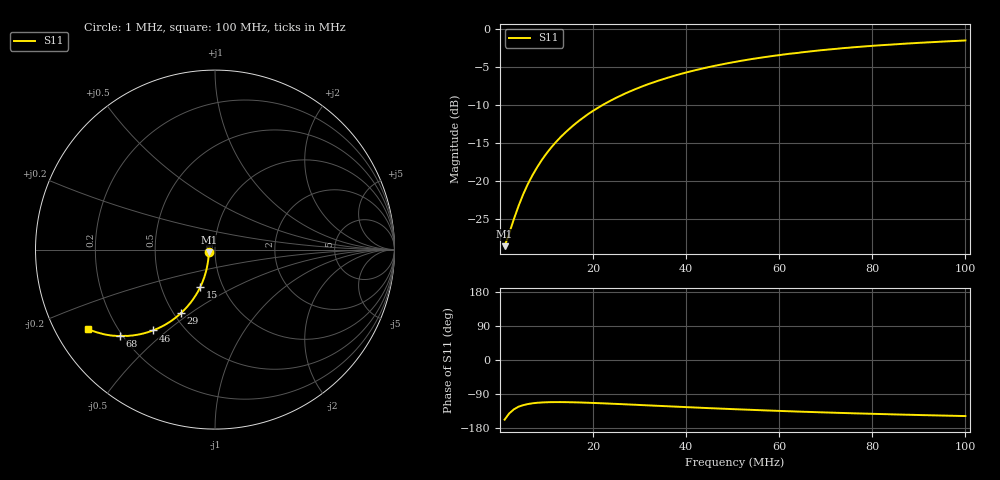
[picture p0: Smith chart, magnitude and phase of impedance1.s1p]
# Hz S RI R 50.0
! written by SimSmith version 18.3b
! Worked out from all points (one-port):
!   100 points, 1 MHz to 100 MHz, reference 50 ohm
!   lowest |S11| = -28.5 dB at 1 MHz (marker M1), VSWR 1.08, Z = 46.6 - j1.35 ohm
!   |S11| at or under -10 dB: start of sweep to 22.1 MHz
!   S11 on the Smith chart (normalised r, x): 1 MHz: 0.93, -0.03; 15 MHz: 0.79, -0.34; 29 MHz: 0.55, -0.46; 46 MHz: 0.34, -0.45; 68 MHz: 0.19, -0.38; 100 MHz: 0.10, -0.28
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1000000  -0.0347 -0.0145
2000000  -0.0355 -0.0289
3000000  -0.0366 -0.0433
4000000  -0.0377 -0.0578
5000000  -0.0401 -0.0719
6000000  -0.0425 -0.0861
7000000  -0.0451 -0.1001
8000000  -0.0482 -0.1139
9000000  -0.0518 -0.1279
1e7  -0.0559 -0.1414
1.2e7  -0.065 -0.1681
1.4e7  -0.0752 -0.1939
1.5e7  -0.081 -0.2063
1.7e7  -0.0933 -0.231
2e7  -0.1146 -0.2654
2.3e7  -0.1374 -0.2974
2.6e7  -0.1621 -0.3262
2.9e7  -0.1882 -0.3528
3.4e7  -0.2339 -0.3905
3.9e7  -0.281 -0.4204
4.6e7  -0.3467 -0.4507
5.1e7  -0.3916 -0.4652
5.6e7  -0.4349 -0.4748
6.3e7  -0.4913 -0.481
6.8e7  -0.5287 -0.4817
7.6e7  -0.5829 -0.478
8.8e7  -0.651 -0.4631
1e8  -0.7079 -0.4432
